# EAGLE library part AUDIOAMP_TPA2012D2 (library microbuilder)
TPA2012D2 2.1W/CH Stereo Class-D Audio Amp 2.1W/Ch into 4 Ohm at 5V 1.4W/Ch into 8 Ohm at 5V 720mW/Ch into 8 ohm at 3.6V Selectable Gain: 6, 12, 18 or 24 dB Power Supply (PVDD and AVDD): 2.5-5.5V Operating Temperature: -40 to 85°C Digikey (QFN20): 296-17692-1-ND
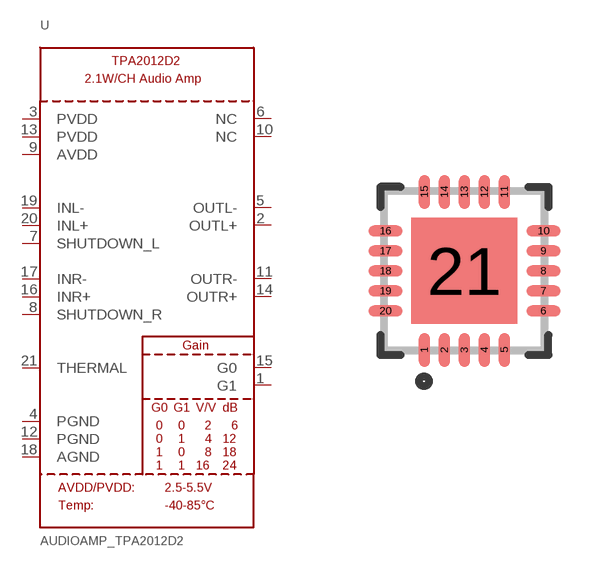
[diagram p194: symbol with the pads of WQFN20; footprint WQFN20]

Designator prefix U

## AUDIOAMP_TPA2012D2  [WQFN20]
1  G1  in
2  OUTL+  out
3  PVDD  pwr
4  PGND  pwr
5  OUTL-  out
6  NC  nc
7  SHUTDOWN_L  in
8  SHUTDOWN_R  in
9  AVDD  pwr
10  NC  nc
11  OUTR-  out
12  PGND  pwr
13  PVDD  pwr
14  OUTR+  out
15  G0  in
16  INR+  in
17  INR-  in
18  AGND  pwr
19  INL-  in
20  INL+  in
21  THERMAL

## Footprint WQFN20 (pad centres in mm)
20-PWQFN 4.0x4.0mm 0.5mm pitch Source: http://www.ti.com/lit/ds/symlink/tpa2012d2.pdf
smd 0.28 x 0.85: 1 -1,-1.975; 2 -0.5,-1.975; 3 0,-1.975; 4 0.5,-1.975; 5 1,-1.975; 11 1,1.975; 12 0.5,1.975; 13 0,1.975; 14 -0.5,1.975; 15 -1,1.975
smd 0.85 x 0.28: 6 1.975,-1; 7 1.975,-0.5; 8 1.975,0; 9 1.975,0.5; 10 1.975,1; 16 -1.975,1; 17 -1.975,0.5; 18 -1.975,0; 19 -1.975,-0.5; 20 -1.975,-1
smd 2.65 x 2.65: 21 0,0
